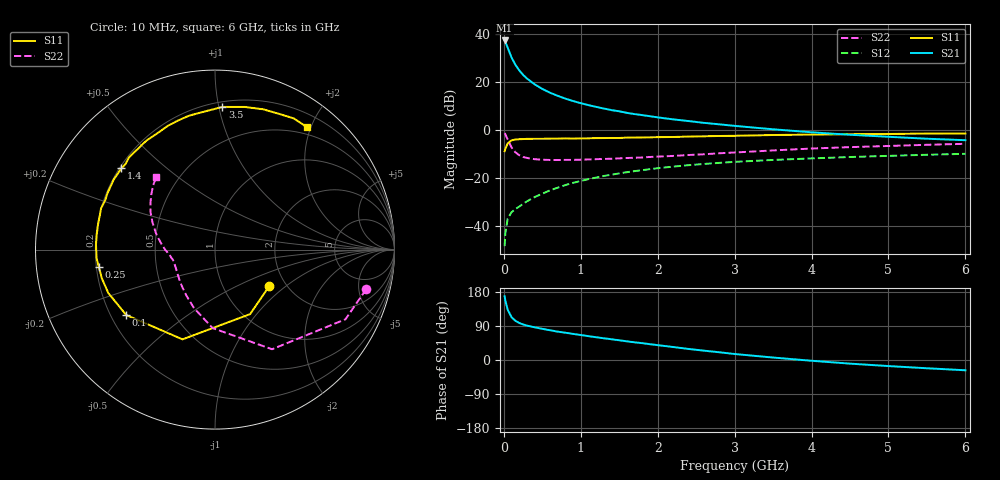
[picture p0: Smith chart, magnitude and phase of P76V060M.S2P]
! SIEMENS Small Signal Semiconductors
! BFP196
! Si NPN RF Bipolar Junction Transistor in SOT143
! VCE = 6 V  IC = 60 mA
! Common Emitter S-Parameters:  May  1996
# GHz  S  MA  R  50
!  f  S11  S21  S12  S22
! GHz  MAG  ANG  MAG  ANG  MAG  ANG  MAG  ANG
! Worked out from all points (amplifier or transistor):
!   36 points, 10 MHz to 6 GHz, reference 50 ohm
!   highest |S21| = 37.5 dB at 10 MHz (marker M1)
!   |S21| within 3 dB of that: start of sweep to 49.69 MHz
!   unconditionally stable (mu >= 1): 453.7 MHz to 4.48 GHz
!   at 250 MHz: K = 0.84, MSG = 26.9 dB, |S12| = -30.8 dB
!   at 1.4 GHz: K = 1.09, MAG = 11.7 dB, |S12| = -18.6 dB
!   at 6 GHz: K = 0.98, MSG = 2.8 dB, |S12| = -9.8 dB
!   S11 on the Smith chart (normalised r, x): 10 MHz: 1.64, -0.77; 100 MHz: 0.26, -0.31; 250 MHz: 0.21, -0.07; 1.4 GHz: 0.21, +0.36; 3.5 GHz: 0.24, +1.03; 6 GHz: 0.38, +1.93
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0.01  0.3641 -33.8  75.01 168.0  0.0038 81.3  0.8709 -14.7
0.02  0.4092 -61.4  69.64 156.3  0.0072 71.2  0.8241 -28.1
0.05  0.5318 -109.9  52.95 132.7  0.0142 54.2  0.6397 -60.2
0.1  0.6143 -143.6  33.15 113.0  0.0195 48.2  0.4376 -91.7
0.15  0.642 -157.9  23.3 103.5  0.0227 49.2  0.3464 -109.7
0.2  0.6505 -165.8  17.87 97.7  0.0255 52.6  0.3018 -121.9
0.25  0.6547 -171.6  14.35 93.8  0.029 54.2  0.2769 -131.2
0.3  0.6616 -175.9  12.06 90.8  0.0328 56.9  0.2644 -137.5
0.4  0.6637 177.5  9.116 86.3  0.0403 60.2  0.2488 -146.9
0.5  0.6643 172.7  7.299 82.3  0.0474 61.7  0.2423 -153.2
0.6  0.6665 167.9  6.087 78.5  0.0556 62.4  0.24 -157.3
0.7  0.6693 163.5  5.242 74.8  0.0633 62.7  0.2395 -160.5
0.9  0.6704 155.8  4.076 68.9  0.0799 61.4  0.2408 -165.5
1.1  0.6795 149.0  3.351 62.9  0.0953 59.9  0.2461 -168.8
1.4  0.6905 139.0  2.635 54.8  0.1179 56.4  0.2546 -172.8
1.7  0.7049 129.7  2.174 46.6  0.1404 52.3  0.2668 -177.3
2.2  0.7232 116.4  1.689 34.3  0.174 45.0  0.2911 176.3
2.8  0.7594 101.1  1.33 20.4  0.2086 36.1  0.3307 166.9
3.5  0.7959 87.0  1.048 6.5  0.24 26.2  0.3793 156.6
4.5  0.8267 71.0  0.805 -9.6  0.2763 14.3  0.4444 144.0
5.5  0.8525 59.0  0.666 -21.8  0.3078 3.7  0.4973 133.8
6  0.8532 53.3  0.62 -27.1  0.3223 -2.0  0.5214 128.8
